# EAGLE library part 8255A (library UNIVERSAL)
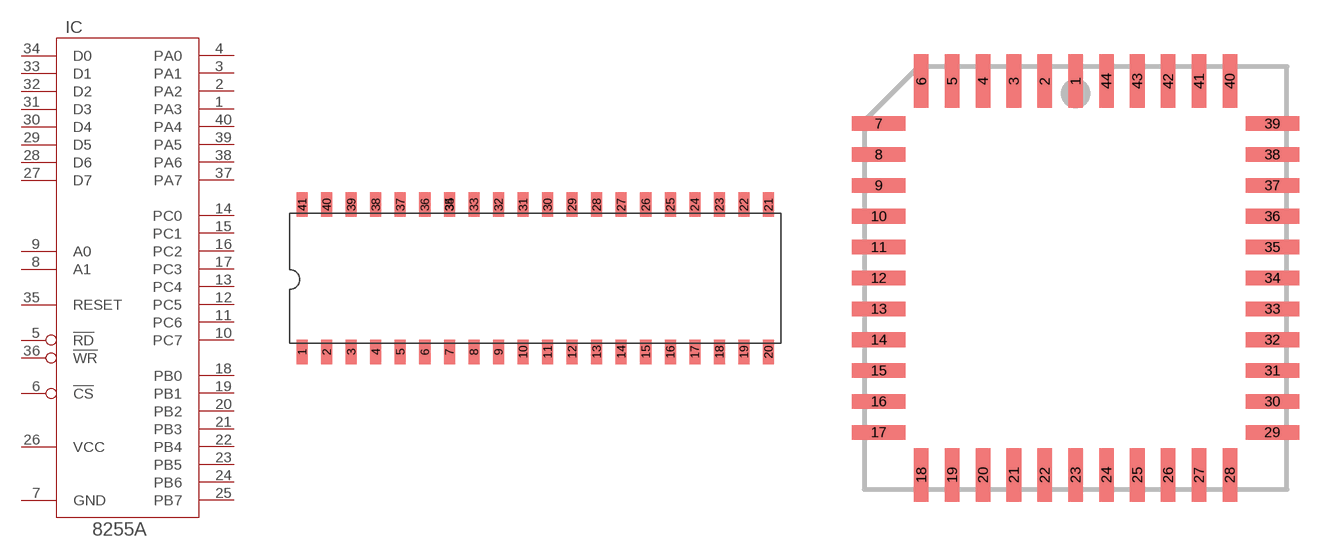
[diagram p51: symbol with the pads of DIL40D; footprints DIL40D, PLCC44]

Designator prefix IC

## 8255ADIPDIP, 8255APLCCDIP  [DIL40D]
1  PA3
2  PA2
3  PA1
4  PA0
5  !RD  in
6  !CS  in
7  GND  pwr
8  A1  in
9  A0  in
10  PC7
11  PC6
12  PC5
13  PC4
14  PC0
15  PC1
16  PC2
17  PC3
18  PB0
19  PB1
20  PB2
21  PB3
22  PB4
23  PB5
24  PB6
25  PB7
26  VCC  pwr
27  D7
28  D6
29  D5
30  D4
31  D3
32  D2
33  D1
34  D0
35  RESET  in
36  !WR  in
37  PA7
38  PA6
39  PA5
40  PA4

## 8255APLCC44  [PLCC44]
2  PA3
3  PA2
4  PA1
5  PA0
6  !RD  in
7  !CS  in
8  GND  pwr
9  A1  in
10  A0  in
11  PC7
13  PC6
14  PC5
15  PC4
16  PC0
17  PC1
18  PC2
19  PC3
20  PB0
21  PB1
22  PB2
24  PB3
25  PB4
26  PB5
27  PB6
28  PB7
29  VCC  pwr
30  D7
31  D6
32  D5
33  D4
35  D3
36  D2
37  D1
38  D0
39  RESET  in
40  !WR  in
41  PA7
42  PA6
43  PA5
44  PA4

## Footprint DIL40D (pad centres in mm)
smd 1.27 x 2.54: 1 0,0; 2 2.54,0; 3 5.08,0; 4 7.62,0; 5 10.16,0; 6 12.7,0; 7 15.24,0; 8 17.78,0; 9 20.32,0; 10 22.86,0; 11 25.4,0; 12 27.94,0; 13 30.48,0; 14 33.02,0; 15 35.56,0; 16 38.1,0; 17 40.64,0; 18 43.18,0; 19 45.72,0; 20 48.26,0; 21 48.26,15.24; 22 45.72,15.24; 23 43.18,15.24; 24 40.64,15.24; 25 38.1,15.24; 26 35.56,15.24; 27 33.02,15.24; 28 30.48,15.24; 29 27.94,15.24; 30 25.4,15.24; 31 22.86,15.24; 32 20.32,15.24; 33 17.78,15.24; 34 15.24,15.24; 35 15.24,15.24; 36 12.7,15.24; 37 10.16,15.24; 38 7.62,15.24; 39 5.08,15.24; 40 2.54,15.24; 41 0,15.24

## Footprint PLCC44 (pad centres in mm)
smd 0.6 x 2.2: 1 0,8.1; 2 -1.27,8.1; 3 -2.54,8.1; 4 -3.81,8.1; 5 -5.08,8.1; 6 -6.35,8.1; 18 -6.35,-8.1; 19 -5.08,-8.1; 20 -3.81,-8.1; 21 -2.54,-8.1; 22 -1.27,-8.1; 23 0,-8.1; 24 1.27,-8.1; 25 2.54,-8.1; 26 3.81,-8.1; 27 5.08,-8.1; 28 6.35,-8.1; 40 6.35,8.1; 41 5.08,8.1; 42 3.81,8.1; 43 2.54,8.1; 44 1.27,8.1
smd 2.2 x 0.6: 7 -8.1,6.35; 8 -8.1,5.08; 9 -8.1,3.81; 10 -8.1,2.54; 11 -8.1,1.27; 12 -8.1,0; 13 -8.1,-1.27; 14 -8.1,-2.54; 15 -8.1,-3.81; 16 -8.1,-5.08; 17 -8.1,-6.35; 29 8.1,-6.35; 30 8.1,-5.08; 31 8.1,-3.81; 32 8.1,-2.54; 33 8.1,-1.27; 34 8.1,0; 35 8.1,1.27; 36 8.1,2.54; 37 8.1,3.81; 38 8.1,5.08; 39 8.1,6.35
